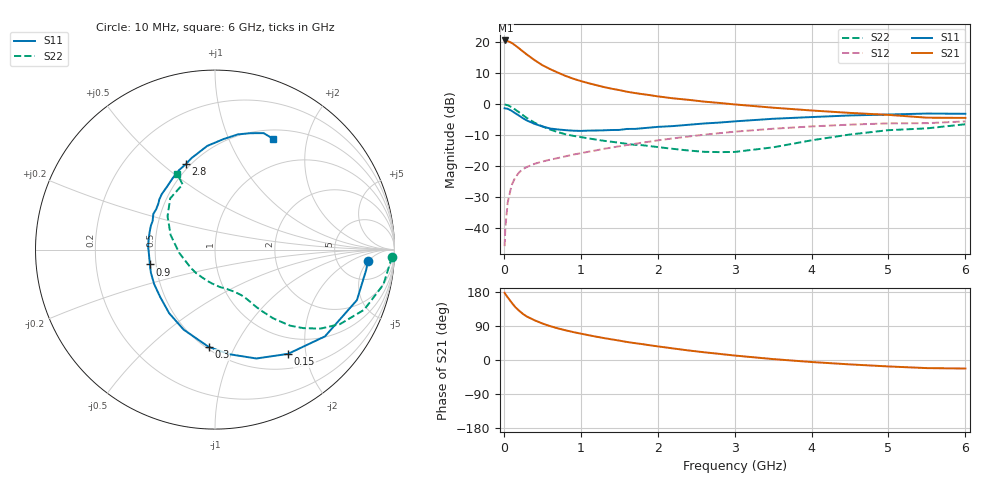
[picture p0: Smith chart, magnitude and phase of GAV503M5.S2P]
! Infineon Technologies  Discrete & RF Semiconductors
! BF775
! Si NPN RF Bipolar Junction Transistor in SOT23
! VCE = 0.5 V  IC = 3.5 mA
! Common Emitter S-Parameters:  May  1996
# GHz  S  MA  R  50
!  f  S11  S21  S12  S22
! GHz  MAG  ANG  MAG  ANG  MAG  ANG  MAG  ANG
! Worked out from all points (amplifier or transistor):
!   36 points, 10 MHz to 6 GHz, reference 50 ohm
!   highest |S21| = 20.5 dB at 20 MHz (marker M1)
!   |S21| within 3 dB of that: start of sweep to 220.5 MHz
!   unconditionally stable (mu >= 1): 766.9 MHz to end of sweep
!   at 250 MHz: K = 0.44, MSG = 18.9 dB, |S12| = -20.9 dB
!   at 1.4 GHz: K = 1.22, MAG = 6.6 dB, |S12| = -14.0 dB
!   at 6 GHz: K = 1.09, MAG = -1.2 dB, |S12| = -5.6 dB
!   S11 on the Smith chart (normalised r, x): 10 MHz: 11, -5; 150 MHz: 0.72, -1.69; 300 MHz: 0.52, -0.79; 900 MHz: 0.46, -0.09; 2.8 GHz: 0.47, +0.60; 6 GHz: 0.61, +1.47
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0.01  0.8545 -4.1  10.58 177.3  0.0051 86.4  0.9852 -2.3
0.02  0.8498 -7.7  10.62 173.9  0.0103 83.9  0.9774 -4.7
0.05  0.8393 -19.6  10.38 165.3  0.0258 79.0  0.9584 -11.7
0.1  0.7804 -38.3  9.73 151.8  0.0487 69.0  0.8957 -22.0
0.15  0.7092 -55.0  8.803 139.2  0.0661 61.0  0.8108 -30.8
0.2  0.649 -69.2  7.877 129.8  0.0793 55.7  0.7347 -36.8
0.25  0.5887 -82.1  7.03 121.3  0.0897 51.2  0.6593 -41.6
0.3  0.5434 -93.7  6.287 114.6  0.0967 48.5  0.595 -45.4
0.4  0.4789 -111.4  5.107 104.8  0.1087 45.2  0.5009 -49.8
0.5  0.4369 -125.8  4.246 96.4  0.1183 43.6  0.4361 -52.4
0.6  0.4035 -139.3  3.669 89.5  0.1265 43.0  0.3885 -54.5
0.7  0.3897 -150.4  3.223 83.6  0.1344 43.0  0.3533 -55.9
0.9  0.372 -167.2  2.569 73.8  0.1527 43.2  0.3075 -58.5
1.1  0.3731 177.3  2.173 65.5  0.1701 43.6  0.2793 -61.9
1.3  0.3771 165.0  1.883 57.9  0.1895 43.5  0.2557 -65.8
1.6  0.397 149.9  1.582 47.6  0.2184 42.9  0.2281 -73.3
2.2  0.4414 127.1  1.237 30.5  0.2797 38.9  0.1895 -95.1
2.8  0.5025 109.0  1.043 16.2  0.339 32.8  0.1679 -129.1
3.5  0.5791 94.3  0.874 2.4  0.3999 24.0  0.2004 -174.8
4.5  0.6549 78.7  0.72 -11.6  0.4658 11.2  0.3231 144.9
5.5  0.7032 67.3  0.603 -21.4  0.4918 -1.7  0.4056 116.4
6  0.697 62.6  0.598 -22.5  0.5256 -5.3  0.4726 116.6
